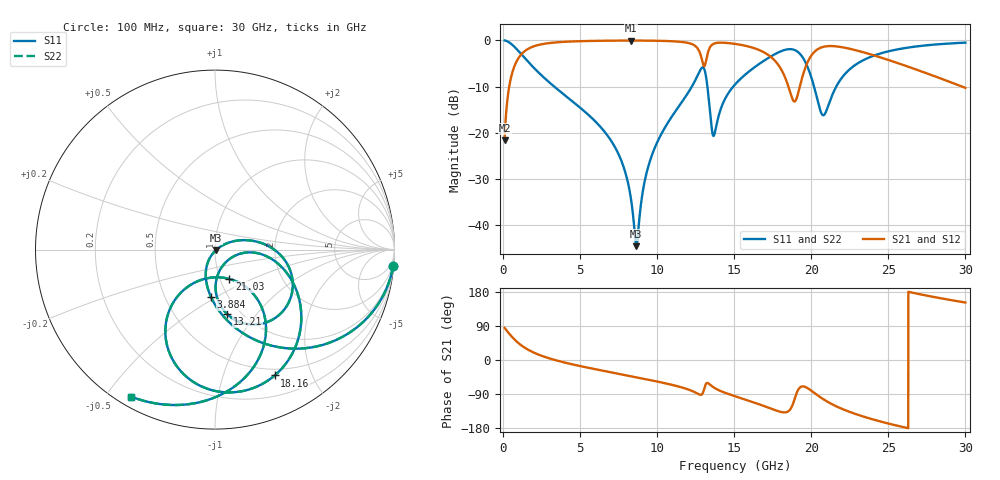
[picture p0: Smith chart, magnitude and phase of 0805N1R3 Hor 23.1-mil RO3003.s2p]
# GHz S MA R 50
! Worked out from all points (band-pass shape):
!   3201 points, 100 MHz to 30 GHz, reference 50 ohm
!   highest |S21| = -0.05 dB at 8.313 GHz (marker M1); lowest = -21.6 dB at 100 MHz (marker M2)
!   |S21| within 3 dB of the highest: 1.178 GHz to 12.81 GHz (11.63 GHz wide, 166 % of centre); 13.26 GHz to 17.16 GHz (3.898 GHz wide, 25.6 % of centre)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
!   lowest |S11| = -44.5 dB at 8.65 GHz (marker M3), VSWR 1.01, Z = 50.4 - j0.447 ohm
!   |S11| at or under -10 dB: 3.315 GHz to 12.25 GHz (8.937 GHz wide, 115 % of centre); 13.26 GHz to 14.94 GHz (1.679 GHz wide, 11.9 % of centre); 20.18 GHz to 21.62 GHz (1.443 GHz wide, 6.9 % of centre)
!   |S22| runs from -44.5 to 0.0 dB; largest |S21 - S12| = 0
!   S11 on the Smith chart (normalised r, x): 100 MHz: 1, -22; 3.884 GHz: 0.83, -0.47; 13.21 GHz: 0.87, -0.72; 18.16 GHz: 0.42, -1.50; 21.03 GHz: 1.11, -0.37; 30 GHz: 0.04, -0.58
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0.1  0.9965 -5.3  0.08321 84.7  0.08321 84.7  0.9965 -5.3
0.47375  0.9296 -24.2  0.3682 65.8  0.3682 65.8  0.9296 -24.2
1.025031  0.7572 -46.2  0.6521 43.7  0.6521 43.7  0.7572 -46.2
2.155625  0.474 -73.1  0.8784 16.7  0.8784 16.7  0.474 -73.1
3.884219  0.2644 -94.9  0.9613 -5.6  0.9613 -5.6  0.2644 -94.9
5.089563  0.1816 -105.7  0.9796 -16.8  0.9796 -16.8  0.1816 -105.7
7.304031  0.06781 -120.7  0.9926 -34.8  0.9926 -34.8  0.06781 -120.7
8.313156  0.01861 -115.3  0.9939 -42.8  0.9939 -42.8  0.01861 -115.3
8.649531  0.005932 -48.4  0.9938 -45.5  0.9938 -45.5  0.005932 -48.4
9.256875  0.03366 28.2  0.9925 -50.5  0.9925 -50.5  0.03366 28.2
10.06978  0.08336 27.2  0.9882 -57.4  0.9882 -57.4  0.08336 27.2
12.76078  0.464 -21.5  0.7404 -91.4  0.7404 -91.4  0.464 -21.5
13.20928  0.3658 -79.3  0.6456 -61.1  0.6456 -61.1  0.3658 -79.3
13.67647  0.09298 -41.0  0.9192 -72.6  0.9192 -72.6  0.09298 -41.0
15.05  0.3326 -10.4  0.9147 -95.5  0.9147 -95.5  0.3326 -10.4
18.16147  0.776 -64.6  0.4464 -138.0  0.4464 -138.0  0.776 -64.6
18.937  0.7835 -91.2  0.2183 -100.8  0.2183 -100.8  0.7835 -91.2
20.03956  0.3801 -128.2  0.6976 -82.1  0.6976 -82.1  0.3801 -128.2
21.03  0.1822 -63.8  0.8637 -109.6  0.8637 -109.6  0.1822 -63.8
22.42222  0.4742 -54.0  0.8153 -135.9  0.8153 -135.9  0.4742 -54.0
25.01978  0.7611 -80.6  0.6118 -167.9  0.6118 -167.9  0.7611 -80.6
30  0.9434 -119.7  0.306 151.7  0.306 151.7  0.9434 -119.7
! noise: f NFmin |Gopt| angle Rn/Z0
0.1  0.001201  0.9524  1.444  0.005665
3.417  0.00751  0.7455  19.2  0.005769
6.743  0.01312  0.7211  36.15  0.008447
10.06  0.02101  0.7434  52.34  0.01331
13.39  0.1238  0.9373  68.49  0.3011
16.7  0.07426  0.8772  83.2  0.07333
20.03  0.195  0.9431  97.97  0.3305
23.35  0.08859  0.8627  111.1  0.04477
26.67  0.08964  0.85  123.5  0.0292
30  0.1086  0.8648  135.6  0.02541
